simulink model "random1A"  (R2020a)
settings: Solver=VariableStepDiscrete  StartTime=0.0  StopTime=1000  RelTol=1e-3  EnableMultiTasking=on

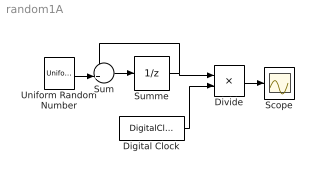
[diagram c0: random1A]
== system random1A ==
  Digital Clock : DigitalClock
  Divide : Product  Inputs=*/
  Scope : Scope
  Sum : Sum  Inputs=++|
  Summe : UnitDelay  SampleTime=-1  HasFrameUpgradeWarning=on
  Uniform Random Number : UniformRandomNumber  Minimum=0  SampleTime=1
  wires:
  Sum/1 -> Summe/1
  Summe/1 -> Sum/1, Divide/1
  Uniform Random Number/1 -> Sum/2
  Digital Clock/1 -> Divide/2
  Divide/1 -> Scope/1
